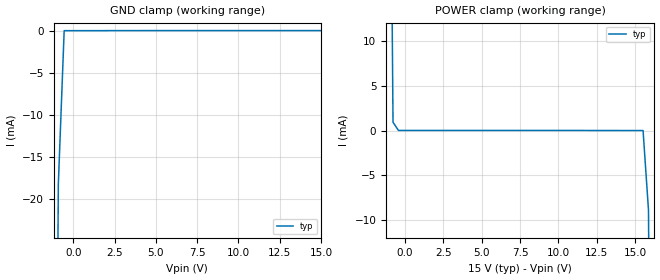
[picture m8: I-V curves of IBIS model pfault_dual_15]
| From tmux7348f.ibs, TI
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| pfault_dual_15
[Model]   pfault_dual_15
Model_type   Input
Vinl = 0.8
Vinh = 1.3
|   typ   min   max
C_comp   1.008417e-11   NA   NA
[Voltage Range]   15   NA   NA
[Temperature Range]   27   NA   NA
[Power Clamp Reference]   15   NA   NA
[GND Clamp Reference]   0   NA   NA
[GND Clamp]
|   Voltage   I(typ)   I(min)   I(max)
-20V      -33.83A    NA         NA
-1.263V   -122.3mA   NA         NA
-909.1mV  -18.23mA   NA         NA
-555.6mV  -854.4nA   NA         NA
15V       9.991uA    NA         NA
[POWER Clamp]
|   Voltage   I(typ)   I(min)   I(max)
-5V       1.413A     NA         NA
-1.111V   74.1mA     NA         NA
-757.6mV  925.7uA    NA         NA
-404mV    9.994uA    NA         NA
15.51V    -348.1nA   NA         NA
15.86V    -8.923mA   NA         NA
16.21V    -106mA     NA         NA
30V       -5.735A    NA         NA
